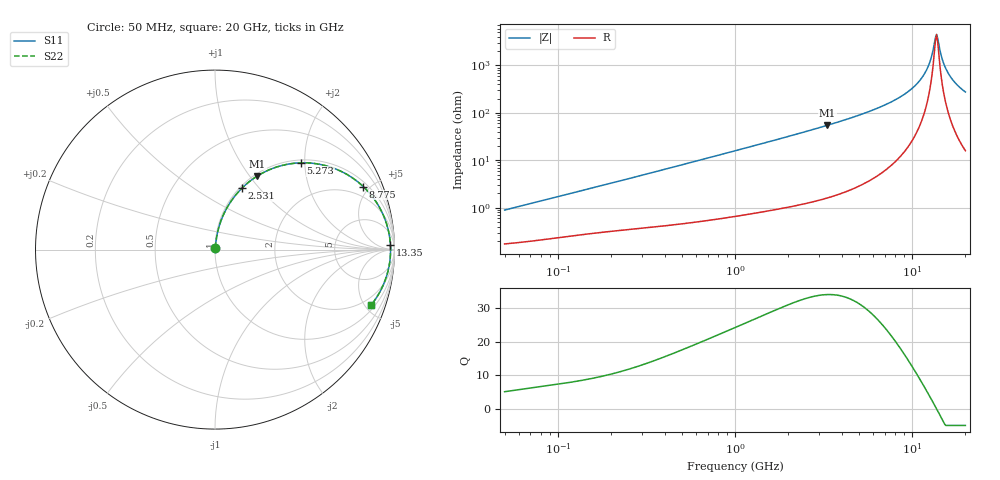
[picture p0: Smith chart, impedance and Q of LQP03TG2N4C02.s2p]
!Murata Part Number: LQP03TG2N4C02
!These Parameters are Measured in Series Mode Connection
!  o--[Z]--o
!Port1  Port2
!  o-------o
!Freq. Start=50[MHz] Stop=20[GHz], 401[Steps]
# Hz S RI R 50
!Freq.(Hz) S11(Real) S11(Imag) S21(Real) S21(Imag) S12(Real) S12(Imag) S22(Real) S22(Imag)
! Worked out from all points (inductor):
!   401 points, 50 MHz to 20 GHz, reference 50 ohm
!   read as one part in series: L = 2.76 nH near 51.52 MHz
!   highest Q = 34.1 at 3.314 GHz (marker M1), where L = 2.62 nH
!   self-resonance near 13.55 GHz
!   S11 on the Smith chart (normalised r, x): 50 MHz: 1.00, +0.02; 2.531 GHz: 1.02, +0.81; 5.273 GHz: 1.06, +1.91; 8.775 GHz: 1.26, +4.57; 13.35 GHz: 37, +44; 20 GHz: 1.32, -5.50
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5e7  0.0018 0.00872  0.9982 -0.00872  0.9982 -0.00872  0.0018 0.00872
1.364002e8  0.00321 0.0227  0.9968 -0.0227  0.9968 -0.0227  0.00321 0.0227
3.721004e8  0.00754 0.0592  0.9925 -0.0592  0.9925 -0.0592  0.00754 0.0592
1e9  0.0305 0.1525  0.9695 -0.1525  0.9695 -0.1525  0.0305 0.1525
2.531158e9  0.1497 0.342  0.8503 -0.342  0.8503 -0.342  0.1497 0.342
2.728004e9  0.1702 0.3612  0.8298 -0.3612  0.8298 -0.3612  0.1702 0.3612
3.314454e9  0.2361 0.4102  0.7639 -0.4102  0.7639 -0.4102  0.2361 0.4102
5.273168e9  0.4786 0.4835  0.5214 -0.4835  0.5214 -0.4835  0.4786 0.4835
7.442007e9  0.7172 0.4287  0.2828 -0.4287  0.2828 -0.4287  0.7172 0.4287
8.774992e9  0.8257 0.3515  0.1743 -0.3515  0.1743 -0.3515  0.8257 0.3515
1.034674e10  0.913 0.2413  0.087 -0.2413  0.087 -0.2413  0.913 0.2413
1.166392e10  0.9556 0.1446  0.0444 -0.1446  0.0444 -0.1446  0.9556 0.1446
1.257102e10  0.9714 0.0795  0.0286 -0.0795  0.0286 -0.0795  0.9714 0.0795
1.334722e10  0.9775 0.026  0.0225 -0.026  0.0225 -0.026  0.9775 0.026
1.354865e10  0.9781 0.0125  0.0219 -0.0125  0.0219 -0.0125  0.9781 0.0125
1.375312e10  0.9783 -0.00103  0.0217 0.00103  0.0217 0.00103  0.9783 -0.00103
1.396067e10  0.9782 -0.0145  0.0218 0.0145  0.0218 0.0145  0.9782 -0.0145
1.504638e10  0.9718 -0.0817  0.0282 0.0817  0.0282 0.0817  0.9718 -0.0817
1.573793e10  0.9636 -0.1212  0.0364 0.1212  0.0364 0.1212  0.9636 -0.1212
1.646126e10  0.9521 -0.1597  0.0479 0.1597  0.0479 0.1597  0.9521 -0.1597
1.800918e10  0.9203 -0.2328  0.0797 0.2328  0.0797 0.2328  0.9203 -0.2328
2e10  0.8698 -0.3087  0.1302 0.3087  0.1302 0.3087  0.8698 -0.3087
